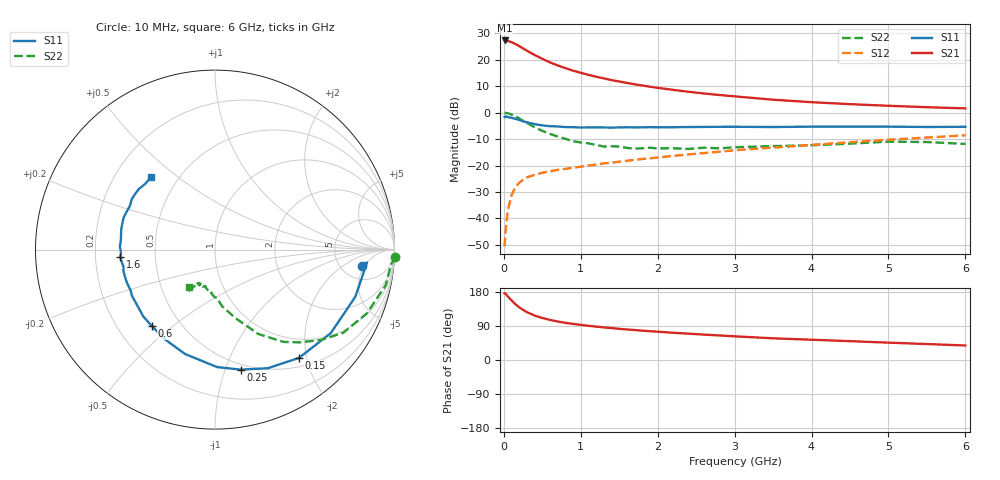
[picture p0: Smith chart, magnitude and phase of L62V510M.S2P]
!  INFINEON TECHNOLOGIES Small Signal Semiconductors
! BFR380L3 , Si-NPN RF-Transistor in TSLP-3-1
!  Vce=2.5 V,  Ic=10 mA
! Common Emitter S-Parameters:  07. March 2005
#  GHz  S  MA  R  50
! f  S11  S21  S12  S22
! GHz  Mag  Ang  Mag  Ang  Mag  Ang  Mag  Ang
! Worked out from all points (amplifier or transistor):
!   36 points, 10 MHz to 6 GHz, reference 50 ohm
!   highest |S21| = 27.2 dB at 10 MHz (marker M1)
!   |S21| within 3 dB of that: start of sweep to 250.6 MHz
!   unconditionally stable (mu >= 1): 2.15 GHz to 4.761 GHz
!   at 250 MHz: K = 0.26, MSG = 24.8 dB, |S12| = -25.4 dB
!   at 1.4 GHz: K = 0.89, MSG = 15.6 dB, |S12| = -18.9 dB
!   at 6 GHz: K = 0.96, MSG = 5.1 dB, |S12| = -8.6 dB
!   S11 on the Smith chart (normalised r, x): 10 MHz: 7.88, -4.35; 150 MHz: 0.64, -1.87; 250 MHz: 0.45, -1.13; 600 MHz: 0.35, -0.43; 1.6 GHz: 0.31, -0.03; 6 GHz: 0.35, +0.41
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0.01  0.8232 -6.2  23.01 175.8  0.003 85.0  1.006 -2.4
0.02  0.8502 -4.8  22.79 175.5  0.0052 91.8  0.9837 -4.9
0.05  0.8249 -18.5  22.53 168.1  0.0137 82.2  0.9718 -11.8
0.1  0.7957 -35.7  21.3 157.3  0.0276 73.1  0.9176 -22.8
0.15  0.7637 -52.2  19.75 147.4  0.0386 65.9  0.8512 -33.0
0.2  0.7235 -66.0  17.97 139.0  0.0472 61.0  0.7767 -40.4
0.25  0.6839 -77.9  16.31 132.3  0.0537 56.2  0.6989 -47.7
0.3  0.6546 -89.0  14.72 126.3  0.0598 53.1  0.6407 -53.4
0.4  0.6052 -106.0  12.24 117.3  0.0667 49.0  0.5288 -62.8
0.5  0.5726 -119.1  10.35 110.9  0.0728 47.4  0.4511 -68.2
0.6  0.553 -129.4  8.857 105.7  0.0779 46.8  0.3965 -73.6
0.8  0.5328 -144.4  6.904 98.1  0.0865 47.5  0.3189 -82.8
0.9  0.5297 -150.7  6.187 95.2  0.0905 48.2  0.2881 -85.7
1.1  0.5244 -159.2  5.155 90.2  0.1001 50.0  0.2629 -91.1
1.4  0.519 -169.3  4.112 84.3  0.113 52.4  0.2314 -97.3
1.6  0.5284 -175.7  3.625 80.6  0.1229 53.8  0.2148 -104.5
2.2  0.5283 172.3  2.686 71.9  0.1521 57.2  0.212 -109.8
2.8  0.5382 162.3  2.149 64.8  0.1822 59.5  0.2111 -117.4
3.5  0.5333 152.8  1.75 57.2  0.2183 59.7  0.2328 -119.3
4.5  0.5427 145.6  1.443 49.7  0.2758 60.4  0.2593 -121.3
5.5  0.5342 136.6  1.263 42.1  0.3381 58.4  0.2776 -123.2
6  0.5392 131.1  1.199 38.3  0.372 56.8  0.256 -125.1
